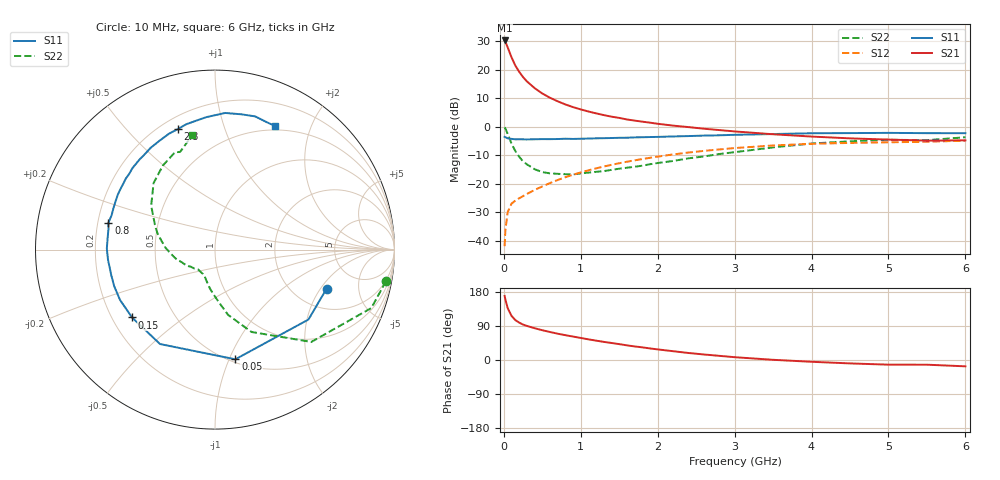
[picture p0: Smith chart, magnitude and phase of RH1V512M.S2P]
! SIEMENS Small Signal Semiconductors
! BFR106
! Si NPN RF Bipolar Junction Transistor in SOT23
! VCE = 1.5 V  IC = 12 mA
! Common Emitter S-Parameters:  August  1996
# GHz  S  MA  R  50
!  f  S11  S21  S12  S22
! GHz  MAG  ANG  MAG  ANG  MAG  ANG  MAG  ANG
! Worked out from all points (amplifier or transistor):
!   36 points, 10 MHz to 6 GHz, reference 50 ohm
!   highest |S21| = 30.2 dB at 10 MHz (marker M1)
!   |S21| within 3 dB of that: start of sweep to 58.02 MHz
!   unconditionally stable (mu >= 1): 436.5 MHz to 2.507 GHz; 4.422 GHz to end of sweep
!   at 250 MHz: K = 0.78, MSG = 20.9 dB, |S12| = -24.4 dB
!   at 1.4 GHz: K = 1.11, MAG = 6.4 dB, |S12| = -13.4 dB
!   at 6 GHz: K = 1.02, MAG = -0.9 dB, |S12| = -4.9 dB
!   S11 on the Smith chart (normalised r, x): 10 MHz: 2.97, -2.29; 50 MHz: 0.53, -1.05; 150 MHz: 0.28, -0.33; 800 MHz: 0.24, +0.12; 2.8 GHz: 0.27, +0.70; 6 GHz: 0.45, +1.50
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0.01  0.6588 -19.3  32.33 169.0  0.008 83.2  0.9687 -10.5
0.02  0.6504 -36.8  30.89 159.8  0.0153 74.8  0.9297 -20.5
0.05  0.6216 -79.5  24.41 136.9  0.0315 57.2  0.7433 -43.8
0.1  0.6088 -120.2  16.34 116.4  0.0446 45.9  0.502 -66.1
0.15  0.5972 -140.7  11.7 105.2  0.0504 44.1  0.3705 -78.7
0.2  0.5989 -152.1  9.102 98.6  0.0554 45.0  0.2948 -85.7
0.25  0.5975 -160.1  7.36 93.4  0.0603 46.5  0.2449 -92.7
0.3  0.5952 -166.1  6.197 89.9  0.0658 48.9  0.2175 -97.6
0.4  0.5989 -174.7  4.722 83.9  0.0775 52.7  0.1789 -105.6
0.5  0.6027 179.4  3.8 78.6  0.0892 55.1  0.1589 -111.5
0.6  0.6017 173.9  3.198 73.9  0.1021 56.9  0.1512 -116.7
0.7  0.6044 169.2  2.772 69.4  0.1157 58.0  0.1484 -121.9
0.8  0.6122 165.8  2.442 65.5  0.1294 58.3  0.1462 -126.8
1.1  0.616 154.0  1.837 54.5  0.171 58.2  0.1562 -137.6
1.3  0.6256 147.4  1.588 47.8  0.1993 56.7  0.1655 -145.0
1.6  0.6374 138.6  1.332 38.7  0.2416 53.9  0.1899 -155.2
2.2  0.671 122.3  1.039 23.2  0.3243 45.9  0.2494 -175.3
2.8  0.7027 107.2  0.868 11.0  0.3972 36.5  0.3299 164.9
3.5  0.7395 93.8  0.733 0.5  0.4657 25.1  0.4313 145.5
4.5  0.768 78.9  0.621 -9.0  0.5165 9.7  0.5512 121.8
5.5  0.7661 67.9  0.567 -12.4  0.5416 0.3  0.5776 109.7
6  0.7657 64.0  0.573 -16.7  0.566 -6.8  0.6492 101.3
